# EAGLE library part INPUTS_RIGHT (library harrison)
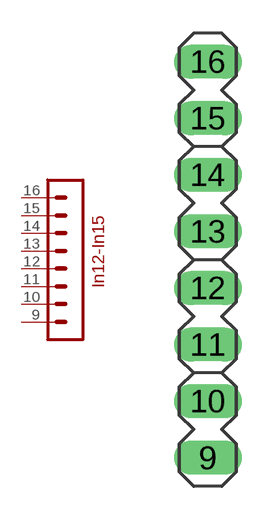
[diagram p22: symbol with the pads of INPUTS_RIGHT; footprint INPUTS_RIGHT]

Designator prefix -

## INPUTS_RIGHT  [INPUTS_RIGHT]
9  P$8  pas
10  P$7  pas
11  P$6  pas
12  P$5  pas
13  P$4  pas
14  P$3  pas
15  P$2  pas
16  P$1  pas

## Footprint INPUTS_RIGHT (pad centres in mm)
drill 1.016 long: 9 0,-6.985; 10 0,-4.445; 11 0,-1.905; 12 0,0.635; 13 0,3.175; 14 0,5.715; 15 0,8.255; 16 0,10.795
